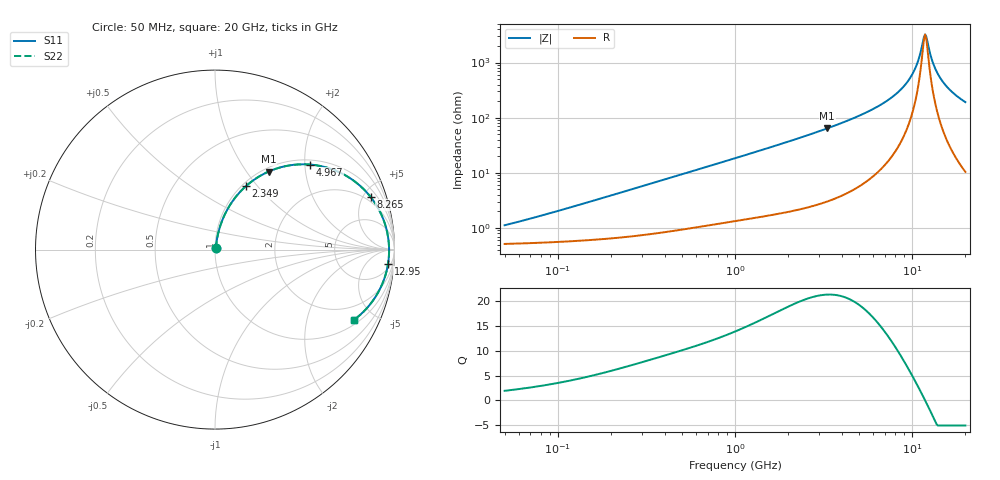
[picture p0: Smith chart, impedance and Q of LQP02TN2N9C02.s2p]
!Murata Part Number: LQP02TN2N9C02
!These Parameters are Measured in Series Mode Connection
!  o--[Z]--o
!Port1  Port2
!  o-------o
!Freq. Start=50[MHz] Stop=20[GHz], 401[Steps]
# Hz S RI R 50
!Freq.(Hz) S11(Real) S11(Imag) S21(Real) S21(Imag) S12(Real) S12(Imag) S22(Real) S22(Imag)
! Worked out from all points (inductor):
!   401 points, 50 MHz to 20 GHz, reference 50 ohm
!   read as one part in series: L = 3.11 nH near 83.2 MHz
!   highest Q = 21.2 at 3.314 GHz (marker M1), where L = 3.07 nH
!   self-resonance near 11.84 GHz
!   S11 on the Smith chart (normalised r, x): 50 MHz: 1.01, +0.02; 2.349 GHz: 1.04, +0.87; 4.967 GHz: 1.11, +2.13; 8.265 GHz: 1.56, +5.64; 12.95 GHz: 8, -21; 20 GHz: 1.21, -3.82
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5e7  0.0052 0.00984  0.9948 -0.00984  0.9948 -0.00984  0.0052 0.00984
1.364002e8  0.00655 0.0261  0.9934 -0.0261  0.9934 -0.0261  0.00655 0.0261
3.721004e8  0.0128 0.0687  0.9872 -0.0687  0.9872 -0.0687  0.0128 0.0687
1e9  0.0444 0.1729  0.9556 -0.1729  0.9556 -0.1729  0.0444 0.1729
2.348516e9  0.1721 0.3532  0.8279 -0.3532  0.8279 -0.3532  0.1721 0.3532
2.728004e9  0.2196 0.3905  0.7804 -0.3905  0.7804 -0.3905  0.2196 0.3905
3.314454e9  0.2987 0.4347  0.7013 -0.4347  0.7013 -0.4347  0.2987 0.4347
4.966507e9  0.5311 0.4737  0.4689 -0.4737  0.4689 -0.4737  0.5311 0.4737
6.125241e9  0.6763 0.4383  0.3237 -0.4383  0.3237 -0.4383  0.6763 0.4383
7.442007e9  0.8063 0.3572  0.1937 -0.3572  0.1937 -0.3572  0.8063 0.3572
8.264682e9  0.8666 0.2938  0.1334 -0.2938  0.1334 -0.2938  0.8666 0.2938
9.316812e9  0.9215 0.2065  0.0785 -0.2065  0.0785 -0.2065  0.9215 0.2065
1.019291e10  0.9502 0.1328  0.0498 -0.1328  0.0498 -0.1328  0.9502 0.1328
1.082228e10  0.9625 0.081  0.0375 -0.081  0.0375 -0.081  0.9625 0.081
1.149051e10  0.969 0.0278  0.031 -0.0278  0.031 -0.0278  0.969 0.0278
1.183995e10  0.97 0.001  0.03 -0.001  0.03 -0.001  0.97 0.001
1.220001e10  0.9695 -0.0259  0.0305 0.0259  0.0305 0.0259  0.9695 -0.0259
1.295331e10  0.9641 -0.0792  0.0359 0.0792  0.0359 0.0792  0.9641 -0.0792
1.396067e10  0.9491 -0.1444  0.0509 0.1444  0.0509 0.1444  0.9491 -0.1444
1.527346e10  0.9197 -0.2182  0.0803 0.2182  0.0803 0.2182  0.9197 -0.2182
1.721783e10  0.8637 -0.3057  0.1363 0.3057  0.1363 0.3057  0.8637 -0.3057
2e10  0.7734 -0.3923  0.2266 0.3923  0.2266 0.3923  0.7734 -0.3923
